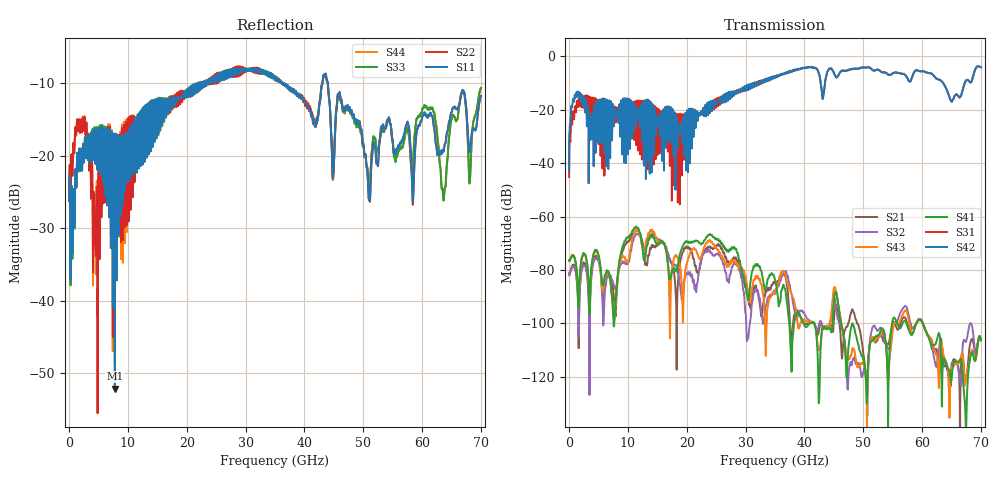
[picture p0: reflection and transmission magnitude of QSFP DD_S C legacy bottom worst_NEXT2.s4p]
! AWR Design Environment (8415) Thu Dec 20 15:43:00 2018
! Document = 'CHANNEL TEST'
! nPorts: 4, nXvals: 7001
# HZ S DB R 50
!Freq DBS11 AngS11 DBS12 AngS12 DBS13 AngS13 DBS14 AngS14
!	DBS21 AngS21 DBS22 AngS22 DBS23 AngS23 DBS24 AngS24
!	DBS31 AngS31 DBS32 AngS32 DBS33 AngS33 DBS34 AngS34
!	DBS41 AngS41 DBS42 AngS42 DBS43 AngS43 DBS44 AngS44
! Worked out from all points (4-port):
!   7000 points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, 10 MHz to 70 GHz, reference 50 ohm
!   strongest paths, dB at 10 MHz, 17.51 GHz, 35.01 GHz, 52.51 GHz, 70 GHz:
!     S42: -42.7, -23.1, -7.5, -5.0, -4.0
!     S31: -45.2, -30.1, -7.6, -5.0, -4.0
!     S41: -76.5, -80.3, -83.8, -104.4, -106.2
!     S43: -76.3, -79.7, -88.9, -105.0, -106.4
!     S32: -82.0, -77.6, -88.0, -102.5, -106.1
!     S21: -81.3, -77.7, -84.8, -105.6, -105.9
!   lowest |S11| = -52.1 dB at 7.78 GHz (marker M1), VSWR 1.00, Z = 49.9 - j0.242 ohm
!   |S11| at or under -10 dB: start of sweep to 21.78 GHz; 36.28 GHz to 43.07 GHz (6.789 GHz wide, 17.1 % of centre); 43.97 GHz to end of sweep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
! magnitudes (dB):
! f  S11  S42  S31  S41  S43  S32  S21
! 10 MHz  -26.3  -42.7  -45.2  -76.5  -76.3  -82.0  -81.3
! 1.3 GHz  -22.2  -13.2  -16.9  -80.5  -80.5  -83.7  -83.3
! 7.78 GHz  -52.1  -19.5  -18.9  -96.3  -96.3  -86.8  -94.6
! 11.41 GHz  -16.4  -21.5  -27.1  -63.8  -64.9  -66.4  -65.0
! 17.26 GHz  -12.6  -19.0  -22.5  -83.1  -88.9  -77.0  -76.6
! 63.65 GHz  -19.4  -10.2  -10.2  -113.2  -111.9  -113.2  -115.7
! 70 GHz  -11.8  -4.0  -4.0  -106.2  -106.4  -106.1  -105.9
